TYPE ST_TopologyData :
STRUCT
	iOwnPhysicalAddr 	: UINT;
	iOwnAutoIncAddr		: UINT;
	stPhysicalAddr		: ST_PortAddr;
	stAutoIncAddr		: ST_PortAddr;
	iPortDelay			: ARRAY [0..2] OF UDINT; (* EC_AD, EC_DB, EC_BC *)
	iReserved			: ARRAY [0..7] OF UDINT;
END_STRUCT
END_TYPE
